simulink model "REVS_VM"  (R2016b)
settings: Solver=ode3  StartTime=REVS.sim_start_time_secs  StopTime=Inf  FixedStep=REVS.sim_step_time_secs  MaxStep=REVS.sim_step_time_secs  EnableMultiTasking=on
StopFcn:
  | postproc_datalog;
  | postproc_audit;
  | postproc_result;
model workspace (MATLAB code in the model file):
  other statements: REVS_setup_variants
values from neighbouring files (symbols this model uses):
  accessory = class_accessory_data    [class_test_data.m]
  battery = class_battery_data    [class_accessory_data.m]    (also in class_REVS_electric.m = class_REVS_battery)
  brake = struct(	'max_torque_Nm',[], 						'proportion_norm',1.0, 						'inertia_kgm2',0.0)    [class_REVS_drive_axle.m]
  engine = class_engine_data    [class_test_data.m]
  final_drive = struct(	'gear_ratio',[], 								'efficiency_norm',[], 								'inertia_kgm2',[] )    [class_REVS_drive_axle.m]
  gear = class_REVS_gearbox    [class_REVS_AT_transmission.m]
  tire = struct(	'radius_m',[], 						'rolling_resistance_coefficient',0, 						'vehicle_weight_norm',1.0,  						'wheel_slip_torque_Nm',[],  						'inertia_kgm2',0.0)    [class_REVS_drive_axle.m]
  torque_converter = class_REVS_torque_converter    [class_REVS_AT_transmission.m]
  transmission = class_transmission_data    [class_test_data.m]
  vehicle = class_vehicle_data    [class_test_data.m]
undefined symbols (not defined in the file or in its folder): alternator, ambient, controls, convert, DelayTimeSecs, drive_cycle, driver, electric, gear_strategy, InitialCondition, InitialValue, LoadSource, LookupStructure, MultiplyPosInputs, Normalize, NumPhases, REVS, SpeedSource, starter, tableshift, UpperSaturationLimit, Value, VerboseLevel, VerboseSignal
libraries: simulink x153
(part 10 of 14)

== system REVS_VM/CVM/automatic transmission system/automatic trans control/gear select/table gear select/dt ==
  Clock : Clock
  Memory1 : Memory
  Sum : Sum  Inputs=|-+
  dt : Outport
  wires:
  Clock/1 -> Sum/2, Memory1/1
  Memory1/1 -> Sum/1
  Sum/1 -> dt/1

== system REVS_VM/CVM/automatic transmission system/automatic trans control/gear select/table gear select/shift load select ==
  system_bus : Inport
  Bus Selector : BusSelector  OutputSignals=driver.driver_acl_norm,engine.eng_load_norm,engine.eng_load_Nm
  Constant1 : Constant  Value=LoadSource
  Constant2 : Constant  Value=0
  Multiport Switch : MultiPortSwitch  DataPortOrder=Specify indices  DataPortIndices={enum_load_source.driver_acl_norm, enum_load_source.engine_load_norm,enum_load_source.driver_acl_pct, enum_load_source.engine_load_pct, enum_load_source.engine_load_Nm}  DataPortForDefault=Additional data port
  acl norm to % : Gain  Gain=100
  load norm to % : Gain  Gain=100
  load : Outport
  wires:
  load norm to %/1 -> Multiport Switch/5
  acl norm to %/1 -> Multiport Switch/4
  Bus Selector/2 -> load norm to %/1, Multiport Switch/3  "<eng_load_norm>"
  Bus Selector/1 -> Multiport Switch/2, acl norm to %/1  "<driver_acl_norm>"
  system_bus/1 -> Bus Selector/1
  Multiport Switch/1 -> load/1
  Constant1/1 -> Multiport Switch/1
  Bus Selector/3 -> Multiport Switch/6  "<eng_load_Nm>"
  Constant2/1 -> Multiport Switch/7

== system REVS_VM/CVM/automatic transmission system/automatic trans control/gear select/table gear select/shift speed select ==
  system_bus : Inport
  Bus Selector : BusSelector  OutputSignals=vehicle.chassis.veh_spd_mps,trans.trans_spd_out_radps,engine.eng_spd_radps,trans.core.trans_spd_in_radps
  Constant : Constant  Value=0
  Constant1 : Constant  Value=SpeedSource
  Multiport Switch : MultiPortSwitch  DataPortOrder=Specify indices  DataPortIndices="{enum_speed_source.vehicle_speed_mph, enum_speed_source.gearbox_output_rpm, enum_speed_source.vehicle_wheel_rpm, enum_speed_source.engine_speed_rpm, enum_speed_source.gearbox_input_rpm, enum_speed_source.gearbox_input_radps, enum_speed_source.gearbox_output_radps, enum_speed_source.engine_speed_radps, enum_speed_source.vehicle_speed_mps,  enum_speed_source.vehicle_speed_kmh}"  DataPortForDefault=Additional data port
  Subsystem : Subsystem
  mps2kmh : Gain  Gain=convert.mps2kmh
  mps2mph : Gain  Gain=convert.mps2mph
  radps2rpm{,1..3} (4 alike) : Gain  Gain=convert.radps2rpm
  spd : Outport
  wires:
  mps2kmh/1 -> Multiport Switch/11
  Subsystem/1(wheel_spd_radps) -> radps2rpm1/1
  system_bus/1 -> Bus Selector/1
  radps2rpm1/1 -> Multiport Switch/4
  mps2mph/1 -> Multiport Switch/2
  Bus Selector/2 -> radps2rpm/1, Multiport Switch/8  "<trans_spd_out_radps>"
  radps2rpm/1 -> Multiport Switch/3
  Multiport Switch/1 -> spd/1
  Constant1/1 -> Multiport Switch/1
  Bus Selector/1 -> Subsystem/1(veh_spd_mps), Multiport Switch/10, mps2kmh/1, mps2mph/1  "<veh_spd_mps>"
  Constant/1 -> Multiport Switch/12
  Bus Selector/3 -> Multiport Switch/9, radps2rpm2/1  "<eng_spd_radps>"
  radps2rpm2/1 -> Multiport Switch/5
  Bus Selector/4 -> Multiport Switch/7, radps2rpm3/1  "<trans_spd_in_radps>"
  radps2rpm3/1 -> Multiport Switch/6

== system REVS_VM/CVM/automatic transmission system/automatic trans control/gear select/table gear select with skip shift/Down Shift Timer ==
  Bool : Inport
  Constant1 : Constant
  Integrator1 : Integrator  ExternalReset=level  UpperSaturationLimit=1  LowerSaturationLimit=0  ZeroCross=off
  Logical Operator : Logic  Operator=NOT  AllPortsSameDT=off  OutDataTypeStr=boolean
  Timer : Outport
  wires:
  Bool/1 -> Logical Operator/1
  Constant1/1 -> Integrator1/1
  Integrator1/1 -> Timer/1
  Logical Operator/1 -> Integrator1/2

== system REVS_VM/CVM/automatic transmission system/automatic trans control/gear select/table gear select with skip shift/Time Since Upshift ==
  Bool : Inport
  Constant1 : Constant
  Integrator1 : Integrator  ExternalReset=level  UpperSaturationLimit=1  LowerSaturationLimit=0  ZeroCross=off
  Timer : Outport
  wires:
  Bool/1 -> Integrator1/2
  Integrator1/1 -> Timer/1
  Constant1/1 -> Integrator1/1

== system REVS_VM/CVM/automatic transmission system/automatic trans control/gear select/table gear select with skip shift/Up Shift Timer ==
  Bool : Inport
  Constant1 : Constant
  Integrator1 : Integrator  ExternalReset=level  UpperSaturationLimit=1  LowerSaturationLimit=0  ZeroCross=off
  Logical Operator : Logic  Operator=NOT  AllPortsSameDT=off  OutDataTypeStr=boolean
  Timer : Outport
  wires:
  Logical Operator/1 -> Integrator1/2
  Integrator1/1 -> Timer/1
  Constant1/1 -> Integrator1/1
  Bool/1 -> Logical Operator/1

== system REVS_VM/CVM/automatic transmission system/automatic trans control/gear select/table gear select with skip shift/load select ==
  system_bus : Inport
  Bus Selector : BusSelector  OutputSignals=driver.driver_acl_norm,engine.eng_load_norm,engine.eng_load_Nm
  Constant1 : Constant  Value=LoadSource
  Constant2 : Constant  Value=0
  Multiport Switch : MultiPortSwitch  DataPortOrder=Specify indices  DataPortIndices={enum_load_source.driver_acl_norm, enum_load_source.engine_load_norm,enum_load_source.driver_acl_pct, enum_load_source.engine_load_pct, enum_load_source.engine_load_Nm}  DataPortForDefault=Additional data port
  acl norm to % : Gain  Gain=100
  load norm to % : Gain  Gain=100
  load : Outport
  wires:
  load norm to %/1 -> Multiport Switch/5
  acl norm to %/1 -> Multiport Switch/4
  Bus Selector/2 -> load norm to %/1, Multiport Switch/3  "<eng_load_norm>"
  Bus Selector/1 -> Multiport Switch/2, acl norm to %/1  "<driver_acl_norm>"
  system_bus/1 -> Bus Selector/1
  Multiport Switch/1 -> load/1
  Constant1/1 -> Multiport Switch/1
  Bus Selector/3 -> Multiport Switch/6  "<eng_load_Nm>"
  Constant2/1 -> Multiport Switch/7

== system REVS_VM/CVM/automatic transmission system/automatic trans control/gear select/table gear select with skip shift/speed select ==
  system_bus : Inport
  Bus Selector : BusSelector  OutputSignals=vehicle.chassis.veh_spd_mps,trans.trans_spd_out_radps,engine.eng_spd_radps,trans.core.trans_spd_in_radps
  Constant : Constant  Value=0
  Constant1 : Constant  Value=SpeedSource
  Multiport Switch : MultiPortSwitch  DataPortOrder=Specify indices  DataPortIndices="{enum_speed_source.vehicle_speed_mph, enum_speed_source.gearbox_output_rpm, enum_speed_source.vehicle_wheel_rpm, enum_speed_source.engine_speed_rpm, enum_speed_source.gearbox_input_rpm, enum_speed_source.gearbox_input_radps, enum_speed_source.gearbox_output_radps, enum_speed_source.engine_speed_radps, enum_speed_source.vehicle_speed_mps,  enum_speed_source.vehicle_speed_kmh}"  DataPortForDefault=Additional data port
  Subsystem : Subsystem
  mps2kmh : Gain  Gain=convert.mps2kmh
  mps2mph : Gain  Gain=convert.mps2mph
  radps2rpm{,1..3} (4 alike) : Gain  Gain=convert.radps2rpm
  spd : Outport
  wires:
  mps2kmh/1 -> Multiport Switch/11
  Subsystem/1(wheel_spd_radps) -> radps2rpm1/1
  system_bus/1 -> Bus Selector/1
  radps2rpm1/1 -> Multiport Switch/4
  mps2mph/1 -> Multiport Switch/2
  Bus Selector/2 -> radps2rpm/1, Multiport Switch/8  "<trans_spd_out_radps>"
  radps2rpm/1 -> Multiport Switch/3
  Multiport Switch/1 -> spd/1
  Constant1/1 -> Multiport Switch/1
  Bus Selector/1 -> Subsystem/1(veh_spd_mps), Multiport Switch/10, mps2kmh/1, mps2mph/1  "<veh_spd_mps>"
  Constant/1 -> Multiport Switch/12
  Bus Selector/3 -> Multiport Switch/9, radps2rpm2/1  "<eng_spd_radps>"
  radps2rpm2/1 -> Multiport Switch/5
  Bus Selector/4 -> Multiport Switch/7, radps2rpm3/1  "<trans_spd_in_radps>"
  radps2rpm3/1 -> Multiport Switch/6

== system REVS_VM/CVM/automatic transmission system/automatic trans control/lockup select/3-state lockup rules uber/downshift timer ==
  trigger_bool : Inport
  Compare To Constant : simulink/Logic and Bit Operations/Compare To Constant  relop=<=  const=transmission.tcc_strategy.downshift_unlock_duration_secs  OutDataTypeStr=boolean
  Constant : Constant
  Integrator1 : Integrator  ExternalReset=level  UpperSaturationLimit=Inf  LowerSaturationLimit=0
  timer_bool : Outport
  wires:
  Compare To Constant/1 -> timer_bool/1
  Constant/1 -> Integrator1/1
  Integrator1/1 -> Compare To Constant/1
  trigger_bool/1 -> Integrator1/2

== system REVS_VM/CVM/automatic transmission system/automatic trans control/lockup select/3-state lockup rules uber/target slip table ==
  bus : Inport
  Bus Selector : BusSelector  OutputSignals=gb.gb_cmd_gear,gb_spd_in_radps,ctrl.gb_line_press_bar
  Lookup : Lookup_n-D  NumberOfTableDimensions=10  BreakpointsForDimension1=LookupStructure.axis_1.breakpoints  BreakpointsForDimension2=LookupStructure.axis_2.breakpoints  BreakpointsForDimension3=LookupStructure.axis_3.breakpoints  BreakpointsForDimension4=LookupStructure.axis_4.breakpoints  BreakpointsForDimension5=LookupStructure.axis_5.breakpoints  BreakpointsForDimension6=LookupStructure.axis_6.breakpoints  BreakpointsForDimension7=LookupStructure.axis_7.breakpoints  BreakpointsForDimension8=LookupStructure.axis_8.breakpoints  BreakpointsForDimension9=LookupStructure.axis_9.breakpoints  BreakpointsForDimension10=LookupStructure.axis_10.breakpoints  IndexSearchMethod=Linear search  BeginIndexSearchUsingPreviousIndexResult=on  Table=LookupStructure.table  DiagnosticForOutOfRangeInput=Warning  InternalRulePriority=Speed  RndMeth=Simplest  SupportTunableTableSize=on  MaximumIndicesForEachDimension=LookupStructure.table_size
  out : Outport
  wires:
  bus/1 -> Bus Selector/1
  Lookup/1 -> out/1

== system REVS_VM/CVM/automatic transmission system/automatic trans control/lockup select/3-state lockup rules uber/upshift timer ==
  trigger_bool : Inport
  Compare To Constant : simulink/Logic and Bit Operations/Compare To Constant  relop=<=  const=transmission.tcc_strategy.upshift_unlock_duration_secs  OutDataTypeStr=boolean
  Constant : Constant
  Integrator1 : Integrator  ExternalReset=level  UpperSaturationLimit=Inf  LowerSaturationLimit=0
  timer_bool : Outport
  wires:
  trigger_bool/1 -> Integrator1/2
  Integrator1/1 -> Compare To Constant/1
  Constant/1 -> Integrator1/1
  Compare To Constant/1 -> timer_bool/1

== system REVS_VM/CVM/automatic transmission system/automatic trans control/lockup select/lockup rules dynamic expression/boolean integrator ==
  bool : Inport
  Constant : Constant  Value=Normalize
  Data Type Conversion2 : DataTypeConversion  OutDataTypeStr=double
  Integrator1 : Integrator  ExternalReset=falling  LimitOutput=on  UpperSaturationLimit=UpperSaturationLimit  LowerSaturationLimit=0
  Switch : Switch  Criteria=u2 > Threshold
  normalize : Gain  Gain=1/UpperSaturationLimit
  out : Outport
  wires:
  Switch/1 -> out/1
  normalize/1 -> Switch/1
  Integrator1/1 -> Switch/3, normalize/1
  Constant/1 -> Switch/2
  bool/1 -> Data Type Conversion2/1
  Data Type Conversion2/1 -> Integrator1/1, Integrator1/2

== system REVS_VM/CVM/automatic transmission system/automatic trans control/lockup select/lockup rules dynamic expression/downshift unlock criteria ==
  bus : Inport
  Bus Creator : BusCreator  Inputs=10
  Bus Creator1 : BusCreator  Inputs=2
  Bus Selector : BusSelector  OutputSignals=var_sigs.var_sig1  OutputAsBus=on
  Data Type Conversion : DataTypeConversion  OutDataTypeStr=double
  Display : Display
  Fcn : Fcn
  Variable {1..10} (10 alike) : Constant  Value=nan
  out : Outport
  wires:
  Data Type Conversion/1 -> Fcn/1
  Bus Selector/1 -> Data Type Conversion/1, Display/1
  Bus Creator1/1 -> Bus Selector/1
  Fcn/1 -> out/1
  bus/1 -> Bus Creator1/1  "system_bus"
  Bus Creator/1 -> Bus Creator1/2  "var_sigs"
  Variable 1/1 -> Bus Creator/1  "var_sig1"
  Variable 2/1 -> Bus Creator/2  "var_sig2"
  Variable 3/1 -> Bus Creator/3  "var_sig3"
  Variable 4/1 -> Bus Creator/4  "var_sig4"
  Variable 5/1 -> Bus Creator/5  "var_sig5"
  Variable 6/1 -> Bus Creator/6  "var_sig6"
  Variable 7/1 -> Bus Creator/7  "var_sig7"
  Variable 8/1 -> Bus Creator/8  "var_sig8"
  Variable 9/1 -> Bus Creator/9  "var_sig9"
  Variable 10/1 -> Bus Creator/10  "var_sig10"

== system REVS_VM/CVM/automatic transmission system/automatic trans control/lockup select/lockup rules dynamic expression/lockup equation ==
  bus : Inport
  Bus Creator : BusCreator  Inputs=10
  Bus Creator1 : BusCreator  Inputs=2
  Bus Selector : BusSelector  OutputSignals=var_sigs.var_sig1  OutputAsBus=on
  Data Type Conversion : DataTypeConversion  OutDataTypeStr=double
  Display : Display
  Fcn : Fcn
  Variable {1..10} (10 alike) : Constant  Value=nan
  out : Outport
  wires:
  Data Type Conversion/1 -> Fcn/1
  Bus Selector/1 -> Data Type Conversion/1, Display/1
  Bus Creator1/1 -> Bus Selector/1
  Fcn/1 -> out/1
  bus/1 -> Bus Creator1/1  "system_bus"
  Bus Creator/1 -> Bus Creator1/2  "var_sigs"
  Variable 1/1 -> Bus Creator/1  "var_sig1"
  Variable 2/1 -> Bus Creator/2  "var_sig2"
  Variable 3/1 -> Bus Creator/3  "var_sig3"
  Variable 4/1 -> Bus Creator/4  "var_sig4"
  Variable 5/1 -> Bus Creator/5  "var_sig5"
  Variable 6/1 -> Bus Creator/6  "var_sig6"
  Variable 7/1 -> Bus Creator/7  "var_sig7"
  Variable 8/1 -> Bus Creator/8  "var_sig8"
  Variable 9/1 -> Bus Creator/9  "var_sig9"
  Variable 10/1 -> Bus Creator/10  "var_sig10"

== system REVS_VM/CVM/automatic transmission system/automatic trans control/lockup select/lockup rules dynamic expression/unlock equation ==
  bus : Inport
  Bus Creator : BusCreator  Inputs=10
  Bus Creator1 : BusCreator  Inputs=2
  Bus Selector : BusSelector  OutputSignals=var_sigs.var_sig1  OutputAsBus=on
  Data Type Conversion : DataTypeConversion  OutDataTypeStr=double
  Display : Display
  Fcn : Fcn
  Variable {1..10} (10 alike) : Constant  Value=nan
  out : Outport
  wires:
  Data Type Conversion/1 -> Fcn/1
  Bus Selector/1 -> Data Type Conversion/1, Display/1
  Bus Creator1/1 -> Bus Selector/1
  Fcn/1 -> out/1
  bus/1 -> Bus Creator1/1  "system_bus"
  Bus Creator/1 -> Bus Creator1/2  "var_sigs"
  Variable 1/1 -> Bus Creator/1  "var_sig1"
  Variable 2/1 -> Bus Creator/2  "var_sig2"
  Variable 3/1 -> Bus Creator/3  "var_sig3"
  Variable 4/1 -> Bus Creator/4  "var_sig4"
  Variable 5/1 -> Bus Creator/5  "var_sig5"
  Variable 6/1 -> Bus Creator/6  "var_sig6"
  Variable 7/1 -> Bus Creator/7  "var_sig7"
  Variable 8/1 -> Bus Creator/8  "var_sig8"
  Variable 9/1 -> Bus Creator/9  "var_sig9"
  Variable 10/1 -> Bus Creator/10  "var_sig10"

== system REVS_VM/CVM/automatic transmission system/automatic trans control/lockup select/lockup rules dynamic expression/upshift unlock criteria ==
  bus : Inport
  Bus Creator : BusCreator  Inputs=10
  Bus Creator1 : BusCreator  Inputs=2
  Bus Selector : BusSelector  OutputSignals=var_sigs.var_sig1  OutputAsBus=on
  Data Type Conversion : DataTypeConversion  OutDataTypeStr=double
  Display : Display
  Fcn : Fcn
  Variable {1..10} (10 alike) : Constant  Value=nan
  out : Outport
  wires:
  Data Type Conversion/1 -> Fcn/1
  Bus Selector/1 -> Data Type Conversion/1, Display/1
  Bus Creator1/1 -> Bus Selector/1
  Fcn/1 -> out/1
  bus/1 -> Bus Creator1/1  "system_bus"
  Bus Creator/1 -> Bus Creator1/2  "var_sigs"
  Variable 1/1 -> Bus Creator/1  "var_sig1"
  Variable 2/1 -> Bus Creator/2  "var_sig2"
  Variable 3/1 -> Bus Creator/3  "var_sig3"
  Variable 4/1 -> Bus Creator/4  "var_sig4"
  Variable 5/1 -> Bus Creator/5  "var_sig5"
  Variable 6/1 -> Bus Creator/6  "var_sig6"
  Variable 7/1 -> Bus Creator/7  "var_sig7"
  Variable 8/1 -> Bus Creator/8  "var_sig8"
  Variable 9/1 -> Bus Creator/9  "var_sig9"
  Variable 10/1 -> Bus Creator/10  "var_sig10"

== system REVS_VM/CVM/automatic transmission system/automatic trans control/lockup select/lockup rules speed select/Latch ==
  On : Inport  PortDimensions=1
  Off : Inport  Port=2  PortDimensions=1
  Combinatorial  Logic : CombinatorialLogic  TruthTable=[0;1;0;0;1;1;(tb==2);(tb>=2)]
  Memory2 : Memory  X0=InitialCondition
  Mux : Mux  Inputs=3
  State : Outport  PortDimensions=1
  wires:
  Off/1 -> Mux/2
  On/1 -> Mux/1
  Memory2/1 -> Mux/3
  Mux/1 -> Combinatorial  Logic/1
  Combinatorial  Logic/1 -> State/1, Memory2/1

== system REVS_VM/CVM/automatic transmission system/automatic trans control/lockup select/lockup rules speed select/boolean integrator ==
  bool : Inport
  Constant : Constant  Value=Normalize
  Data Type Conversion2 : DataTypeConversion  OutDataTypeStr=double
  Integrator1 : Integrator  ExternalReset=falling  LimitOutput=on  UpperSaturationLimit=UpperSaturationLimit  LowerSaturationLimit=0
  Switch : Switch  Criteria=u2 > Threshold
  normalize : Gain  Gain=1/UpperSaturationLimit
  out : Outport
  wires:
  Switch/1 -> out/1
  normalize/1 -> Switch/1
  Integrator1/1 -> Switch/3, normalize/1
  Constant/1 -> Switch/2
  bool/1 -> Data Type Conversion2/1
  Data Type Conversion2/1 -> Integrator1/1, Integrator1/2

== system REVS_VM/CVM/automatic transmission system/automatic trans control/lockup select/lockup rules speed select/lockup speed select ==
  system_bus : Inport
  Bus Selector : BusSelector  OutputSignals=vehicle.chassis.veh_spd_mps,trans.trans_spd_out_radps,engine.eng_spd_radps,trans.core.trans_spd_in_radps
  Constant : Constant  Value=0
  Constant1 : Constant  Value=SpeedSource
  Multiport Switch : MultiPortSwitch  DataPortOrder=Specify indices  DataPortIndices="{enum_speed_source.vehicle_speed_mph, enum_speed_source.gearbox_output_rpm, enum_speed_source.vehicle_wheel_rpm, enum_speed_source.engine_speed_rpm, enum_speed_source.gearbox_input_rpm, enum_speed_source.gearbox_input_radps, enum_speed_source.gearbox_output_radps, enum_speed_source.engine_speed_radps, enum_speed_source.vehicle_speed_mps,  enum_speed_source.vehicle_speed_kmh}"  DataPortForDefault=Additional data port
  Subsystem : Subsystem
  mps2kmh : Gain  Gain=convert.mps2kmh
  mps2mph : Gain  Gain=convert.mps2mph
  radps2rpm{,1..3} (4 alike) : Gain  Gain=convert.radps2rpm
  spd : Outport
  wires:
  mps2kmh/1 -> Multiport Switch/11
  Subsystem/1(wheel_spd_radps) -> radps2rpm1/1
  system_bus/1 -> Bus Selector/1
  radps2rpm1/1 -> Multiport Switch/4
  mps2mph/1 -> Multiport Switch/2
  Bus Selector/2 -> radps2rpm/1, Multiport Switch/8  "<trans_spd_out_radps>"
  radps2rpm/1 -> Multiport Switch/3
  Multiport Switch/1 -> spd/1
  Constant1/1 -> Multiport Switch/1
  Bus Selector/1 -> Subsystem/1(veh_spd_mps), Multiport Switch/10, mps2kmh/1, mps2mph/1  "<veh_spd_mps>"
  Constant/1 -> Multiport Switch/12
  Bus Selector/3 -> Multiport Switch/9, radps2rpm2/1  "<eng_spd_radps>"
  radps2rpm2/1 -> Multiport Switch/5
  Bus Selector/4 -> Multiport Switch/7, radps2rpm3/1  "<trans_spd_in_radps>"
  radps2rpm3/1 -> Multiport Switch/6

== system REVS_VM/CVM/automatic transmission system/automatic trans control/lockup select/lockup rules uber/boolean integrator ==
  bool : Inport
  Constant : Constant  Value=Normalize
  Data Type Conversion2 : DataTypeConversion  OutDataTypeStr=double
  Integrator1 : Integrator  ExternalReset=falling  LimitOutput=on  UpperSaturationLimit=UpperSaturationLimit  LowerSaturationLimit=0
  Switch : Switch  Criteria=u2 > Threshold
  normalize : Gain  Gain=1/UpperSaturationLimit
  out : Outport
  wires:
  Switch/1 -> out/1
  normalize/1 -> Switch/1
  Integrator1/1 -> Switch/3, normalize/1
  Constant/1 -> Switch/2
  bool/1 -> Data Type Conversion2/1
  Data Type Conversion2/1 -> Integrator1/1, Integrator1/2

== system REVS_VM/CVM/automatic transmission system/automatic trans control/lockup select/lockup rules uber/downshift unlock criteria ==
  bus : Inport
  Bus Creator : BusCreator  Inputs=10
  Bus Creator1 : BusCreator  Inputs=2
  Bus Selector : BusSelector  OutputSignals=var_sigs.var_sig1  OutputAsBus=on
  Data Type Conversion : DataTypeConversion  OutDataTypeStr=double
  Display : Display
  Fcn : Fcn
  Variable {1..10} (10 alike) : Constant  Value=nan
  out : Outport
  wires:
  Data Type Conversion/1 -> Fcn/1
  Bus Selector/1 -> Data Type Conversion/1, Display/1
  Bus Creator1/1 -> Bus Selector/1
  Fcn/1 -> out/1
  bus/1 -> Bus Creator1/1  "system_bus"
  Bus Creator/1 -> Bus Creator1/2  "var_sigs"
  Variable 1/1 -> Bus Creator/1  "var_sig1"
  Variable 2/1 -> Bus Creator/2  "var_sig2"
  Variable 3/1 -> Bus Creator/3  "var_sig3"
  Variable 4/1 -> Bus Creator/4  "var_sig4"
  Variable 5/1 -> Bus Creator/5  "var_sig5"
  Variable 6/1 -> Bus Creator/6  "var_sig6"
  Variable 7/1 -> Bus Creator/7  "var_sig7"
  Variable 8/1 -> Bus Creator/8  "var_sig8"
  Variable 9/1 -> Bus Creator/9  "var_sig9"
  Variable 10/1 -> Bus Creator/10  "var_sig10"

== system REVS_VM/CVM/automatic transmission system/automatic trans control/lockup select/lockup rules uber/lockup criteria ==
  bus : Inport
  Bus Creator : BusCreator  Inputs=10
  Bus Creator1 : BusCreator  Inputs=2
  Bus Selector : BusSelector  OutputSignals=var_sigs.var_sig1  OutputAsBus=on
  Data Type Conversion : DataTypeConversion  OutDataTypeStr=double
  Display : Display
  Fcn : Fcn
  Variable {1..10} (10 alike) : Constant  Value=nan
  out : Outport
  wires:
  Data Type Conversion/1 -> Fcn/1
  Bus Selector/1 -> Data Type Conversion/1, Display/1
  Bus Creator1/1 -> Bus Selector/1
  Fcn/1 -> out/1
  bus/1 -> Bus Creator1/1  "system_bus"
  Bus Creator/1 -> Bus Creator1/2  "var_sigs"
  Variable 1/1 -> Bus Creator/1  "var_sig1"
  Variable 2/1 -> Bus Creator/2  "var_sig2"
  Variable 3/1 -> Bus Creator/3  "var_sig3"
  Variable 4/1 -> Bus Creator/4  "var_sig4"
  Variable 5/1 -> Bus Creator/5  "var_sig5"
  Variable 6/1 -> Bus Creator/6  "var_sig6"
  Variable 7/1 -> Bus Creator/7  "var_sig7"
  Variable 8/1 -> Bus Creator/8  "var_sig8"
  Variable 9/1 -> Bus Creator/9  "var_sig9"
  Variable 10/1 -> Bus Creator/10  "var_sig10"

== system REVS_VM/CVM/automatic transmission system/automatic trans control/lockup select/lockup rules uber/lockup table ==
  bus : Inport
  Bus Selector : BusSelector  OutputSignals=gb.gb_cmd_gear,gb_spd_in_radps,ctrl.gb_line_press_bar
  Lookup : Lookup_n-D  NumberOfTableDimensions=10  BreakpointsForDimension1=LookupStructure.axis_1.breakpoints  BreakpointsForDimension2=LookupStructure.axis_2.breakpoints  BreakpointsForDimension3=LookupStructure.axis_3.breakpoints  BreakpointsForDimension4=LookupStructure.axis_4.breakpoints  BreakpointsForDimension5=LookupStructure.axis_5.breakpoints  BreakpointsForDimension6=LookupStructure.axis_6.breakpoints  BreakpointsForDimension7=LookupStructure.axis_7.breakpoints  BreakpointsForDimension8=LookupStructure.axis_8.breakpoints  BreakpointsForDimension9=LookupStructure.axis_9.breakpoints  BreakpointsForDimension10=LookupStructure.axis_10.breakpoints  IndexSearchMethod=Linear search  BeginIndexSearchUsingPreviousIndexResult=on  Table=LookupStructure.table  DiagnosticForOutOfRangeInput=Warning  InternalRulePriority=Speed  RndMeth=Simplest  SupportTunableTableSize=on  MaximumIndicesForEachDimension=LookupStructure.table_size
  out : Outport
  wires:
  bus/1 -> Bus Selector/1
  Lookup/1 -> out/1

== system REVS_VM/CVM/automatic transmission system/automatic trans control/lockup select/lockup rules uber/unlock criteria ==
  bus : Inport
  Bus Creator : BusCreator  Inputs=10
  Bus Creator1 : BusCreator  Inputs=2
  Bus Selector : BusSelector  OutputSignals=var_sigs.var_sig1  OutputAsBus=on
  Data Type Conversion : DataTypeConversion  OutDataTypeStr=double
  Display : Display
  Fcn : Fcn
  Variable {1..10} (10 alike) : Constant  Value=nan
  out : Outport
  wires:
  Data Type Conversion/1 -> Fcn/1
  Bus Selector/1 -> Data Type Conversion/1, Display/1
  Bus Creator1/1 -> Bus Selector/1
  Fcn/1 -> out/1
  bus/1 -> Bus Creator1/1  "system_bus"
  Bus Creator/1 -> Bus Creator1/2  "var_sigs"
  Variable 1/1 -> Bus Creator/1  "var_sig1"
  Variable 2/1 -> Bus Creator/2  "var_sig2"
  Variable 3/1 -> Bus Creator/3  "var_sig3"
  Variable 4/1 -> Bus Creator/4  "var_sig4"
  Variable 5/1 -> Bus Creator/5  "var_sig5"
  Variable 6/1 -> Bus Creator/6  "var_sig6"
  Variable 7/1 -> Bus Creator/7  "var_sig7"
  Variable 8/1 -> Bus Creator/8  "var_sig8"
  Variable 9/1 -> Bus Creator/9  "var_sig9"
  Variable 10/1 -> Bus Creator/10  "var_sig10"

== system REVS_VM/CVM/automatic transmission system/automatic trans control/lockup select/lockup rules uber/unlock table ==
  bus : Inport
  Bus Selector : BusSelector  OutputSignals=gb.gb_cmd_gear,gb_spd_in_radps,ctrl.gb_line_press_bar
  Lookup : Lookup_n-D  NumberOfTableDimensions=10  BreakpointsForDimension1=LookupStructure.axis_1.breakpoints  BreakpointsForDimension2=LookupStructure.axis_2.breakpoints  BreakpointsForDimension3=LookupStructure.axis_3.breakpoints  BreakpointsForDimension4=LookupStructure.axis_4.breakpoints  BreakpointsForDimension5=LookupStructure.axis_5.breakpoints  BreakpointsForDimension6=LookupStructure.axis_6.breakpoints  BreakpointsForDimension7=LookupStructure.axis_7.breakpoints  BreakpointsForDimension8=LookupStructure.axis_8.breakpoints  BreakpointsForDimension9=LookupStructure.axis_9.breakpoints  BreakpointsForDimension10=LookupStructure.axis_10.breakpoints  IndexSearchMethod=Linear search  BeginIndexSearchUsingPreviousIndexResult=on  Table=LookupStructure.table  DiagnosticForOutOfRangeInput=Warning  InternalRulePriority=Speed  RndMeth=Simplest  SupportTunableTableSize=on  MaximumIndicesForEachDimension=LookupStructure.table_size
  out : Outport
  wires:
  bus/1 -> Bus Selector/1
  Lookup/1 -> out/1

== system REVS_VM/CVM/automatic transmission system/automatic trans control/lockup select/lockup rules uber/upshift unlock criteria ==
  bus : Inport
  Bus Creator : BusCreator  Inputs=10
  Bus Creator1 : BusCreator  Inputs=2
  Bus Selector : BusSelector  OutputSignals=var_sigs.var_sig1  OutputAsBus=on
  Data Type Conversion : DataTypeConversion  OutDataTypeStr=double
  Display : Display
  Fcn : Fcn
  Variable {1..10} (10 alike) : Constant  Value=nan
  out : Outport
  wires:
  Data Type Conversion/1 -> Fcn/1
  Bus Selector/1 -> Data Type Conversion/1, Display/1
  Bus Creator1/1 -> Bus Selector/1
  Fcn/1 -> out/1
  bus/1 -> Bus Creator1/1  "system_bus"
  Bus Creator/1 -> Bus Creator1/2  "var_sigs"
  Variable 1/1 -> Bus Creator/1  "var_sig1"
  Variable 2/1 -> Bus Creator/2  "var_sig2"
  Variable 3/1 -> Bus Creator/3  "var_sig3"
  Variable 4/1 -> Bus Creator/4  "var_sig4"
  Variable 5/1 -> Bus Creator/5  "var_sig5"
  Variable 6/1 -> Bus Creator/6  "var_sig6"
  Variable 7/1 -> Bus Creator/7  "var_sig7"
  Variable 8/1 -> Bus Creator/8  "var_sig8"
  Variable 9/1 -> Bus Creator/9  "var_sig9"
  Variable 10/1 -> Bus Creator/10  "var_sig10"

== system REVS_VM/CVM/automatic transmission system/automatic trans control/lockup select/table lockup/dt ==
  Clock : Clock
  Memory1 : Memory
  Sum : Sum  Inputs=|-+
  dt : Outport
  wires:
  Clock/1 -> Sum/2, Memory1/1
  Memory1/1 -> Sum/1
  Sum/1 -> dt/1

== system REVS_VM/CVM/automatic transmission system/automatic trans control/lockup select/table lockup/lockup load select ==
  system_bus : Inport
  Bus Selector : BusSelector  OutputSignals=driver.driver_acl_norm,engine.eng_load_norm,engine.eng_load_Nm
  Constant1 : Constant  Value=LoadSource
  Constant2 : Constant  Value=0
  Multiport Switch : MultiPortSwitch  DataPortOrder=Specify indices  DataPortIndices={enum_load_source.driver_acl_norm, enum_load_source.engine_load_norm,enum_load_source.driver_acl_pct, enum_load_source.engine_load_pct, enum_load_source.engine_load_Nm}  DataPortForDefault=Additional data port
  acl norm to % : Gain  Gain=100
  load norm to % : Gain  Gain=100
  load : Outport
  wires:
  load norm to %/1 -> Multiport Switch/5
  acl norm to %/1 -> Multiport Switch/4
  Bus Selector/2 -> load norm to %/1, Multiport Switch/3  "<eng_load_norm>"
  Bus Selector/1 -> Multiport Switch/2, acl norm to %/1  "<driver_acl_norm>"
  system_bus/1 -> Bus Selector/1
  Multiport Switch/1 -> load/1
  Constant1/1 -> Multiport Switch/1
  Bus Selector/3 -> Multiport Switch/6  "<eng_load_Nm>"
  Constant2/1 -> Multiport Switch/7

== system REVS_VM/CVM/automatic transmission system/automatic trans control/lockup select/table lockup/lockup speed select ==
  system_bus : Inport
  Bus Selector : BusSelector  OutputSignals=vehicle.chassis.veh_spd_mps,trans.trans_spd_out_radps,engine.eng_spd_radps,trans.core.trans_spd_in_radps
  Constant : Constant  Value=0
  Constant1 : Constant  Value=SpeedSource
  Multiport Switch : MultiPortSwitch  DataPortOrder=Specify indices  DataPortIndices="{enum_speed_source.vehicle_speed_mph, enum_speed_source.gearbox_output_rpm, enum_speed_source.vehicle_wheel_rpm, enum_speed_source.engine_speed_rpm, enum_speed_source.gearbox_input_rpm, enum_speed_source.gearbox_input_radps, enum_speed_source.gearbox_output_radps, enum_speed_source.engine_speed_radps, enum_speed_source.vehicle_speed_mps,  enum_speed_source.vehicle_speed_kmh}"  DataPortForDefault=Additional data port
  Subsystem : Subsystem
  mps2kmh : Gain  Gain=convert.mps2kmh
  mps2mph : Gain  Gain=convert.mps2mph
  radps2rpm{,1..3} (4 alike) : Gain  Gain=convert.radps2rpm
  spd : Outport
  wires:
  mps2kmh/1 -> Multiport Switch/11
  Subsystem/1(wheel_spd_radps) -> radps2rpm1/1
  system_bus/1 -> Bus Selector/1
  radps2rpm1/1 -> Multiport Switch/4
  mps2mph/1 -> Multiport Switch/2
  Bus Selector/2 -> radps2rpm/1, Multiport Switch/8  "<trans_spd_out_radps>"
  radps2rpm/1 -> Multiport Switch/3
  Multiport Switch/1 -> spd/1
  Constant1/1 -> Multiport Switch/1
  Bus Selector/1 -> Subsystem/1(veh_spd_mps), Multiport Switch/10, mps2kmh/1, mps2mph/1  "<veh_spd_mps>"
  Constant/1 -> Multiport Switch/12
  Bus Selector/3 -> Multiport Switch/9, radps2rpm2/1  "<eng_spd_radps>"
  radps2rpm2/1 -> Multiport Switch/5
  Bus Selector/4 -> Multiport Switch/7, radps2rpm3/1  "<trans_spd_in_radps>"
  radps2rpm3/1 -> Multiport Switch/6

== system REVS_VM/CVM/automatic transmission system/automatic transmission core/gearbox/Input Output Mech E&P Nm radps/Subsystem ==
  trq_in_Nm : Inport
  spd_in_radps : Inport  Port=2
  iner_in_kgm2 : Inport  Port=3
  trq_out_Nm : Inport  Port=4
  spd_out_radps : Inport  Port=5
  iner_out_kgm2 : Inport  Port=6
  Enable : EnablePort  ZeroCross=off
  Input Mech E&P Nm radps : Subsystem
  Loss_KJ_to_workspace : ToWorkspace  VariableName=audit__mech__gearbox__loss_kJ  SampleTime=-1
  Output Mech E&P Nm radps : Subsystem
  Pos : Saturate  UpperLimit=Inf  LowerLimit=0  ZeroCross=off
  Pos2 : Saturate  UpperLimit=Inf  LowerLimit=0  ZeroCross=off
  Sum : Sum  Inputs=|+-
  Sum1 : Sum  Inputs=-+|
  Sum2 : Sum
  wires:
  Pos2/1 -> Sum2/2
  Pos/1 -> Sum2/1
  trq_in_Nm/1 -> Input Mech E&P Nm radps/1(" trq_Nm")
  spd_in_radps/1 -> Input Mech E&P Nm radps/2(spd_radps)
  trq_out_Nm/1 -> Output Mech E&P Nm radps/1(" trq_Nm")
  spd_out_radps/1 -> Output Mech E&P Nm radps/2(spd_radps)
  iner_in_kgm2/1 -> Input Mech E&P Nm radps/3(iner_kgm2)
  iner_out_kgm2/1 -> Output Mech E&P Nm radps/3(iner_kgm2)
  Input Mech E&P Nm radps/1(pos_kJ) -> Sum/1
  Output Mech E&P Nm radps/1(pos_kJ) -> Sum/2
  Output Mech E&P Nm radps/2(neg_kJ) -> Sum1/2
  Input Mech E&P Nm radps/2(neg_kJ) -> Sum1/1
  Sum/1 -> Pos/1
  Sum1/1 -> Pos2/1
  Sum2/1 -> Loss_KJ_to_workspace/1

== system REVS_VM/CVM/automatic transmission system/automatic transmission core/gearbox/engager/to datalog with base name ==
  Var : Inport
  Constant : Constant  Value=VerboseSignal
  Constant1 : Constant  Value=VerboseLevel
  Relational Operator : RelationalOperator  OutDataTypeStr=boolean  ZeroCross=off
  Subsystem : Subsystem
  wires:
  Constant1/1 -> Relational Operator/2
  Relational Operator/1 -> Subsystem/Enable
  Constant/1 -> Relational Operator/1
  Var/1 -> Subsystem/1(Var)

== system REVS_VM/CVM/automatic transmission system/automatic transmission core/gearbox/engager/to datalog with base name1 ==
  Var : Inport
  Constant : Constant  Value=VerboseSignal
  Constant1 : Constant  Value=VerboseLevel
  Relational Operator : RelationalOperator  OutDataTypeStr=boolean  ZeroCross=off
  Subsystem : Subsystem
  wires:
  Constant1/1 -> Relational Operator/2
  Relational Operator/1 -> Subsystem/Enable
  Constant/1 -> Relational Operator/1
  Var/1 -> Subsystem/1(Var)

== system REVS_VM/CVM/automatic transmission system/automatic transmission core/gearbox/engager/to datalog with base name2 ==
  Var : Inport
  Constant : Constant  Value=VerboseSignal
  Constant1 : Constant  Value=VerboseLevel
  Relational Operator : RelationalOperator  OutDataTypeStr=boolean  ZeroCross=off
  Subsystem : Subsystem
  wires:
  Constant1/1 -> Relational Operator/2
  Relational Operator/1 -> Subsystem/Enable
  Constant/1 -> Relational Operator/1
  Var/1 -> Subsystem/1(Var)

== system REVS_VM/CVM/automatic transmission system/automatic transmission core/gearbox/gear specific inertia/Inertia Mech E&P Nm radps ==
  trq_Nm : Inport
  spd_radps : Inport  Port=2
  Compare To Constant : simulink/Logic and Bit Operations/Compare To Constant  relop=>=  const=1  OutDataTypeStr=boolean
  Constant : Constant  Value=VerboseSignal
  Subsystem : Subsystem
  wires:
  trq_Nm/1 -> Subsystem/1(trq_Nm)
  spd_radps/1 -> Subsystem/2(spd_radps)
  Compare To Constant/1 -> Subsystem/Enable
  Constant/1 -> Compare To Constant/1

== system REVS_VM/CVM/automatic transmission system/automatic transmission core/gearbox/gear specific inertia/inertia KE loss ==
  Var : Inport
  Compare To Constant : simulink/Logic and Bit Operations/Compare To Constant  relop=>=  const=1  OutDataTypeStr=boolean
  Constant : Constant  Value=VerboseSignal
  Subsystem : Subsystem
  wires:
  Constant/1 -> Compare To Constant/1
  Compare To Constant/1 -> Subsystem/Enable
  Var/1 -> Subsystem/1(In1)

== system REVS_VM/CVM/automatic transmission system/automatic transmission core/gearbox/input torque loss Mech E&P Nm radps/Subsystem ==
  trq_Nm : Inport
  spd_radps : Inport  Port=2
  Enable : EnablePort  ZeroCross=off
  Mech Energy Nm radps : Subsystem  TreatAsAtomicUnit=on
  energy_to_workspace : ToWorkspace  VariableName=audit__mech__gearbox__input_torque_loss_kJ  SampleTime=-1
  neg_energy_to_workspace : ToWorkspace  VariableName=audit__mech__gearbox__input_torque_loss_neg_kJ  SampleTime=-1
  pos_energy_to_workspace : ToWorkspace  VariableName=audit__mech__gearbox__input_torque_loss_pos_kJ  SampleTime=-1
  power_to_workspace : ToWorkspace  VariableName=audit__mech__gearbox__input_torque_loss_kW  SampleTime=-1
  speed_to_workspace : ToWorkspace  VariableName=audit__mech__gearbox__input_torque_loss_radps  SampleTime=-1
  torque_to_workspace : ToWorkspace  VariableName=audit__mech__gearbox__input_torque_loss_Nm  SampleTime=-1
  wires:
  Mech Energy Nm radps/1("total_kJ ") -> energy_to_workspace/1
  Mech Energy Nm radps/4(pwr_kW) -> power_to_workspace/1
  Mech Energy Nm radps/2("pos_kJ ") -> pos_energy_to_workspace/1
  Mech Energy Nm radps/3(neg_kJ) -> neg_energy_to_workspace/1
  trq_Nm/1 -> torque_to_workspace/1, Mech Energy Nm radps/1(trq_Nm)
  spd_radps/1 -> speed_to_workspace/1, Mech Energy Nm radps/2(spd_radps)

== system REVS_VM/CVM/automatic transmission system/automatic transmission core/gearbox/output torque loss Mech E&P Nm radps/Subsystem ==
  trq_Nm : Inport
  spd_radps : Inport  Port=2
  Enable : EnablePort  ZeroCross=off
  Mech Energy Nm radps : Subsystem  TreatAsAtomicUnit=on
  energy_to_workspace : ToWorkspace  VariableName=audit__mech__gearbox__output_torque_loss_kJ  SampleTime=-1
  neg_energy_to_workspace : ToWorkspace  VariableName=audit__mech__gearbox__output_torque_loss_neg_kJ  SampleTime=-1
  pos_energy_to_workspace : ToWorkspace  VariableName=audit__mech__gearbox__output_torque_loss_pos_kJ  SampleTime=-1
  power_to_workspace : ToWorkspace  VariableName=audit__mech__gearbox__output_torque_loss_kW  SampleTime=-1
  speed_to_workspace : ToWorkspace  VariableName=audit__mech__gearbox__output_torque_loss_radps  SampleTime=-1
  torque_to_workspace : ToWorkspace  VariableName=audit__mech__gearbox__output_torque_loss_Nm  SampleTime=-1
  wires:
  Mech Energy Nm radps/1("total_kJ ") -> energy_to_workspace/1
  Mech Energy Nm radps/4(pwr_kW) -> power_to_workspace/1
  Mech Energy Nm radps/2("pos_kJ ") -> pos_energy_to_workspace/1
  Mech Energy Nm radps/3(neg_kJ) -> neg_energy_to_workspace/1
  trq_Nm/1 -> torque_to_workspace/1, Mech Energy Nm radps/1(trq_Nm)
  spd_radps/1 -> speed_to_workspace/1, Mech Energy Nm radps/2(spd_radps)

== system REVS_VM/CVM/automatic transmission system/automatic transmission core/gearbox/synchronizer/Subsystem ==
  engage : Inport
  spd_out : Inport  Port=2
  spd_in : Inport  Port=3
  Compare To Constant1 : simulink/Logic and Bit Operations/Compare To Constant  relop=<=  const=1e-3  OutDataTypeStr=boolean  ZeroCross=off
  Compare To Constant2 : simulink/Logic and Bit Operations/Compare To Constant  relop=<=  const=1e-3  OutDataTypeStr=boolean  ZeroCross=off
  Compare To Constant3 : simulink/Logic and Bit Operations/Compare To Constant  relop=>  const=0  OutDataTypeStr=boolean  ZeroCross=off
  Compare To Constant4 : simulink/Logic and Bit Operations/Compare To Constant  relop===  const=1  OutDataTypeStr=boolean
  Logical Operator : Logic  Operator=OR  AllPortsSameDT=off  OutDataTypeStr=boolean
  Logical Operator1 : Logic  Inputs=3  AllPortsSameDT=off  OutDataTypeStr=boolean
  Memory2 : Memory
  lockup : Outport
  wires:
  Compare To Constant3/1 -> Logical Operator1/1
  Logical Operator1/1 -> Memory2/1
  spd_in/1 -> Compare To Constant2/1
  spd_out/1 -> Compare To Constant1/1
  Logical Operator/1 -> lockup/1
  engage/1 -> Compare To Constant4/1, Compare To Constant3/1
  Compare To Constant2/1 -> Logical Operator1/3
  Compare To Constant1/1 -> Logical Operator1/2
  Memory2/1 -> Logical Operator/2
  Compare To Constant4/1 -> Logical Operator/1

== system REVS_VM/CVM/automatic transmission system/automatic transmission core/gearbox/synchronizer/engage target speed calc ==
  engage : Inport
  final_spd_radps : Inport  Port=2
  current_spd_radps : Inport  Port=3
  Compare To Zero : simulink/Logic and Bit Operations/Compare To Zero  relop=>  OutDataTypeStr=boolean
  Fcn : Fcn  Expr=5*(1-u)^3 + .05
  Product1 : Product  Inputs=**//
  Sum2 : Sum  Inputs=|+-
  engage duration : Constant  Value=Value
  engage_accel_radps2 : Outport
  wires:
  current_spd_radps/1 -> Sum2/2
  Product1/1 -> engage_accel_radps2/1
  final_spd_radps/1 -> Sum2/1
  engage/1 -> Fcn/1, Compare To Zero/1
  Compare To Zero/1 -> Product1/1
  engage duration/1 -> Product1/4
  Sum2/1 -> Product1/2
  Fcn/1 -> Product1/3

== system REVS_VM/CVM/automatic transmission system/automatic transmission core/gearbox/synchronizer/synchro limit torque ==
  engage : Inport
  "req_transmit_torque_Nm " : Inport  Port=2
  input_speed_radps : Inport  Port=3
  output_speed_radps : Inport  Port=4
  Compare To Constant2 : simulink/Logic and Bit Operations/Compare To Constant  relop=>  const=0  OutDataTypeStr=boolean
  Compare To Zero : simulink/Logic and Bit Operations/Compare To Zero  relop=>=  OutDataTypeStr=boolean
  Compare To Zero1 : simulink/Logic and Bit Operations/Compare To Zero  relop=<=  OutDataTypeStr=boolean
  Constant : Constant  Value=.1
  Constant1 : Constant  Value=-.1
  Constant2 : Constant  Value=inf
  Constant3 : Constant  Value=-inf
  MinMax : MinMax  Function=max  Inputs=2  ZeroCross=off
  MinMax1 : MinMax  Inputs=2  ZeroCross=off
  Product : Product
  Product1 : Product
  Product2 : Product
  Sum : Sum  Inputs=|+-
  Sum1 : Sum  Inputs=|++
  Sum2 : Sum  Inputs=++|
  lim_transmit_torque_Nm : Outport
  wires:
  Product/1 -> Sum2/2
  Product2/1 -> Sum1/1
  Constant2/1 -> Product/1
  Constant3/1 -> Product2/2
  Compare To Zero1/1 -> Product2/1
  Compare To Zero/1 -> Product/2
  Constant/1 -> Sum2/1
  Constant1/1 -> Sum1/2
  Sum1/1 -> MinMax/2
  Product1/1 -> lim_transmit_torque_Nm/1
  "req_transmit_torque_Nm "/1 -> MinMax1/1
  MinMax/1 -> Product1/2
  engage/1 -> Compare To Constant2/1
  MinMax1/1 -> MinMax/1
  input_speed_radps/1 -> Sum/1
  output_speed_radps/1 -> Sum/2
  Compare To Constant2/1 -> Product1/1
  Sum/1 -> Compare To Zero1/1, Compare To Zero/1
  Sum2/1 -> MinMax1/2

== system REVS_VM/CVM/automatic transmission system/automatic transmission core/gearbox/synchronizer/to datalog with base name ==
  Var : Inport
  Constant : Constant  Value=VerboseSignal
  Constant1 : Constant  Value=VerboseLevel
  Relational Operator : RelationalOperator  OutDataTypeStr=boolean  ZeroCross=off
  Subsystem : Subsystem
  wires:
  Constant1/1 -> Relational Operator/2
  Relational Operator/1 -> Subsystem/Enable
  Constant/1 -> Relational Operator/1
  Var/1 -> Subsystem/1(Var)

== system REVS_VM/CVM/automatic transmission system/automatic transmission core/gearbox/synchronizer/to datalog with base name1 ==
  Var : Inport
  Constant : Constant  Value=VerboseSignal
  Constant1 : Constant  Value=VerboseLevel
  Relational Operator : RelationalOperator  OutDataTypeStr=boolean  ZeroCross=off
  Subsystem : Subsystem
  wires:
  Constant1/1 -> Relational Operator/2
  Relational Operator/1 -> Subsystem/Enable
  Constant/1 -> Relational Operator/1
  Var/1 -> Subsystem/1(Var)

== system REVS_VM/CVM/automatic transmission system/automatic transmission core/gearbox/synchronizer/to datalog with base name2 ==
  Var : Inport
  Constant : Constant  Value=VerboseSignal
  Constant1 : Constant  Value=VerboseLevel
  Relational Operator : RelationalOperator  OutDataTypeStr=boolean  ZeroCross=off
  Subsystem : Subsystem
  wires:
  Constant1/1 -> Relational Operator/2
  Relational Operator/1 -> Subsystem/Enable
  Constant/1 -> Relational Operator/1
  Var/1 -> Subsystem/1(Var)

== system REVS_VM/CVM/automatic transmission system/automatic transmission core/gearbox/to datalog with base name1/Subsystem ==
  Var : Inport
  Enable : EnablePort
  To Workspace : ToWorkspace  VariableName=datalog__gearbox__gear_efficiency_norm  SampleTime=-1
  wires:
  Var/1 -> To Workspace/1

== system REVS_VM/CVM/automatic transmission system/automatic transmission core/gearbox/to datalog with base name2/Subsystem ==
  Var : Inport
  Enable : EnablePort
  To Workspace : ToWorkspace  VariableName=datalog__gearbox__actual_ratio  SampleTime=-1
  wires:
  Var/1 -> To Workspace/1

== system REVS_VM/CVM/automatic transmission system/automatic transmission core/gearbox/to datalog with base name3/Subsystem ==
  Var : Inport
  Enable : EnablePort
  To Workspace : ToWorkspace  VariableName=datalog__gearbox__engage_norm  SampleTime=-1
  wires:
  Var/1 -> To Workspace/1

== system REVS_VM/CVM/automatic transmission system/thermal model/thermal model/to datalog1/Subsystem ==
  In1 : Inport
  Enable : EnablePort
  To Workspace : ToWorkspace  VariableName=datalog__transmission__temperature_C  SampleTime=-1
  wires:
  In1/1 -> To Workspace/1

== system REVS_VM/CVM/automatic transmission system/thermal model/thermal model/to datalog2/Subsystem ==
  In1 : Inport
  Enable : EnablePort
  To Workspace : ToWorkspace  VariableName=datalog__transmission__thermal_loss_power_input_W  SampleTime=-1
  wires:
  In1/1 -> To Workspace/1

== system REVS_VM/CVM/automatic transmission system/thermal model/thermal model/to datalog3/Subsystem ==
  In1 : Inport
  Enable : EnablePort
  To Workspace : ToWorkspace  VariableName=datalog__transmission__thermal_net_power_W  SampleTime=-1
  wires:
  In1/1 -> To Workspace/1

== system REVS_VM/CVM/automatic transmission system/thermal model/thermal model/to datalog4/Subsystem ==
  In1 : Inport
  Enable : EnablePort
  To Workspace : ToWorkspace  VariableName=datalog__transmission__thermal_passive_conduction_power_W  SampleTime=-1
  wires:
  In1/1 -> To Workspace/1

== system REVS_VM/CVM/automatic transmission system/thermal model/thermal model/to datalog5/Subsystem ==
  In1 : Inport
  Enable : EnablePort
  To Workspace : ToWorkspace  VariableName=datalog__transmission__thermal_cooling_conduction_power_W  SampleTime=-1
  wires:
  In1/1 -> To Workspace/1

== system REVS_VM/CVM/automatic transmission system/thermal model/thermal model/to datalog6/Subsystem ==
  In1 : Inport
  Enable : EnablePort
  To Workspace : ToWorkspace  VariableName=datalog__transmission__thermal_conduction_temperature_degC  SampleTime=-1
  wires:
  In1/1 -> To Workspace/1

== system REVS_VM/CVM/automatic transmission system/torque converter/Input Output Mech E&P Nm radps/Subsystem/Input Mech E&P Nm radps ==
  " trq_Nm" : Inport
  spd_radps : Inport  Port=2
  iner_kgm2 : Inport  Port=3
  Compare To Constant : simulink/Logic and Bit Operations/Compare To Constant  relop=>=  const=1  OutDataTypeStr=boolean
  Constant : Constant  Value=VerboseSignal
  Subsystem : Subsystem
  pos_kJ : Outport
  neg_kJ : Outport  Port=2
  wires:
  " trq_Nm"/1 -> Subsystem/1(" trq_Nm")
  spd_radps/1 -> Subsystem/2(spd_radps)
  iner_kgm2/1 -> Subsystem/3(iner_kgm2)
  Compare To Constant/1 -> Subsystem/Enable
  Subsystem/1(pos_kJ) -> pos_kJ/1
  Subsystem/2(neg_kJ) -> neg_kJ/1
  Constant/1 -> Compare To Constant/1

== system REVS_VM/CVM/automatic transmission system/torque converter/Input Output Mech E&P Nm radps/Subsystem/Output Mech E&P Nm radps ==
  " trq_Nm" : Inport
  spd_radps : Inport  Port=2
  iner_kgm2 : Inport  Port=3
  Compare To Constant : simulink/Logic and Bit Operations/Compare To Constant  relop=>=  const=1  OutDataTypeStr=boolean
  Constant : Constant  Value=VerboseSignal
  Subsystem : Subsystem
  pos_kJ : Outport
  neg_kJ : Outport  Port=2
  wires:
  " trq_Nm"/1 -> Subsystem/1(" trq_Nm")
  spd_radps/1 -> Subsystem/2(spd_radps)
  iner_kgm2/1 -> Subsystem/3(iner_kgm2)
  Compare To Constant/1 -> Subsystem/Enable
  Subsystem/1(pos_kJ) -> pos_kJ/1
  Subsystem/2(neg_kJ) -> neg_kJ/1
  Constant/1 -> Compare To Constant/1

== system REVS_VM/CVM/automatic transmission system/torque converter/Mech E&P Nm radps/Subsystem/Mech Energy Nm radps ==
  trq_Nm : Inport
  spd_radps : Inport  Port=2
  Gain : Gain  Gain=-1
  Integrator : Integrator  ZeroCross=off
  Integrator1 : Integrator  ZeroCross=off
  Integrator2 : Integrator  ZeroCross=off
  Mux : Mux  Inputs=2
  Neg : Fcn  Expr=u(1)*(u(1) <= 0)
  Pos : Fcn  Expr=u(1)*(u(1) >= 0)
  calc_Power_kW : Fcn  Expr=u(1)*u(2)/1000
  "total_kJ " : Outport
  "pos_kJ " : Outport  Port=2
  neg_kJ : Outport  Port=3
  pwr_kW : Outport  Port=4
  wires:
  calc_Power_kW/1 -> Pos/1, Neg/1, pwr_kW/1, Integrator/1
  Gain/1 -> neg_kJ/1
  Integrator1/1 -> "pos_kJ "/1
  Integrator2/1 -> Gain/1
  Neg/1 -> Integrator2/1
  Pos/1 -> Integrator1/1
  spd_radps/1 -> Mux/2
  trq_Nm/1 -> Mux/1
  Mux/1 -> calc_Power_kW/1
  Integrator/1 -> "total_kJ "/1

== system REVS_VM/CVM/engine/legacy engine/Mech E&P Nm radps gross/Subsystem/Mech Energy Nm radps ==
  trq_Nm : Inport
  spd_radps : Inport  Port=2
  Gain : Gain  Gain=-1
  Integrator : Integrator  ZeroCross=off
  Integrator1 : Integrator  ZeroCross=off
  Integrator2 : Integrator  ZeroCross=off
  Mux : Mux  Inputs=2
  Neg : Fcn  Expr=u(1)*(u(1) <= 0)
  Pos : Fcn  Expr=u(1)*(u(1) >= 0)
  calc_Power_kW : Fcn  Expr=u(1)*u(2)/1000
  "total_kJ " : Outport
  "pos_kJ " : Outport  Port=2
  neg_kJ : Outport  Port=3
  pwr_kW : Outport  Port=4
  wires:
  calc_Power_kW/1 -> Pos/1, Neg/1, pwr_kW/1, Integrator/1
  Gain/1 -> neg_kJ/1
  Integrator1/1 -> "pos_kJ "/1
  Integrator2/1 -> Gain/1
  Neg/1 -> Integrator2/1
  Pos/1 -> Integrator1/1
  spd_radps/1 -> Mux/2
  trq_Nm/1 -> Mux/1
  Mux/1 -> calc_Power_kW/1
  Integrator/1 -> "total_kJ "/1

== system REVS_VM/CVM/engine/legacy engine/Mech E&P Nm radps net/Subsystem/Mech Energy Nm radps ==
  trq_Nm : Inport
  spd_radps : Inport  Port=2
  Gain : Gain  Gain=-1
  Integrator : Integrator  ZeroCross=off
  Integrator1 : Integrator  ZeroCross=off
  Integrator2 : Integrator  ZeroCross=off
  Mux : Mux  Inputs=2
  Neg : Fcn  Expr=u(1)*(u(1) <= 0)
  Pos : Fcn  Expr=u(1)*(u(1) >= 0)
  calc_Power_kW : Fcn  Expr=u(1)*u(2)/1000
  "total_kJ " : Outport
  "pos_kJ " : Outport  Port=2
  neg_kJ : Outport  Port=3
  pwr_kW : Outport  Port=4
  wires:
  calc_Power_kW/1 -> Pos/1, Neg/1, pwr_kW/1, Integrator/1
  Gain/1 -> neg_kJ/1
  Integrator1/1 -> "pos_kJ "/1
  Integrator2/1 -> Gain/1
  Neg/1 -> Integrator2/1
  Pos/1 -> Integrator1/1
  spd_radps/1 -> Mux/2
  trq_Nm/1 -> Mux/1
  Mux/1 -> calc_Power_kW/1
  Integrator/1 -> "total_kJ "/1

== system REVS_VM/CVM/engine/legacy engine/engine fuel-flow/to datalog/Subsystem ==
  In1 : Inport
  Enable : EnablePort
  To Workspace : ToWorkspace  VariableName=datalog__engine__accel_penalty_gps  SampleTime=-1
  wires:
  In1/1 -> To Workspace/1
